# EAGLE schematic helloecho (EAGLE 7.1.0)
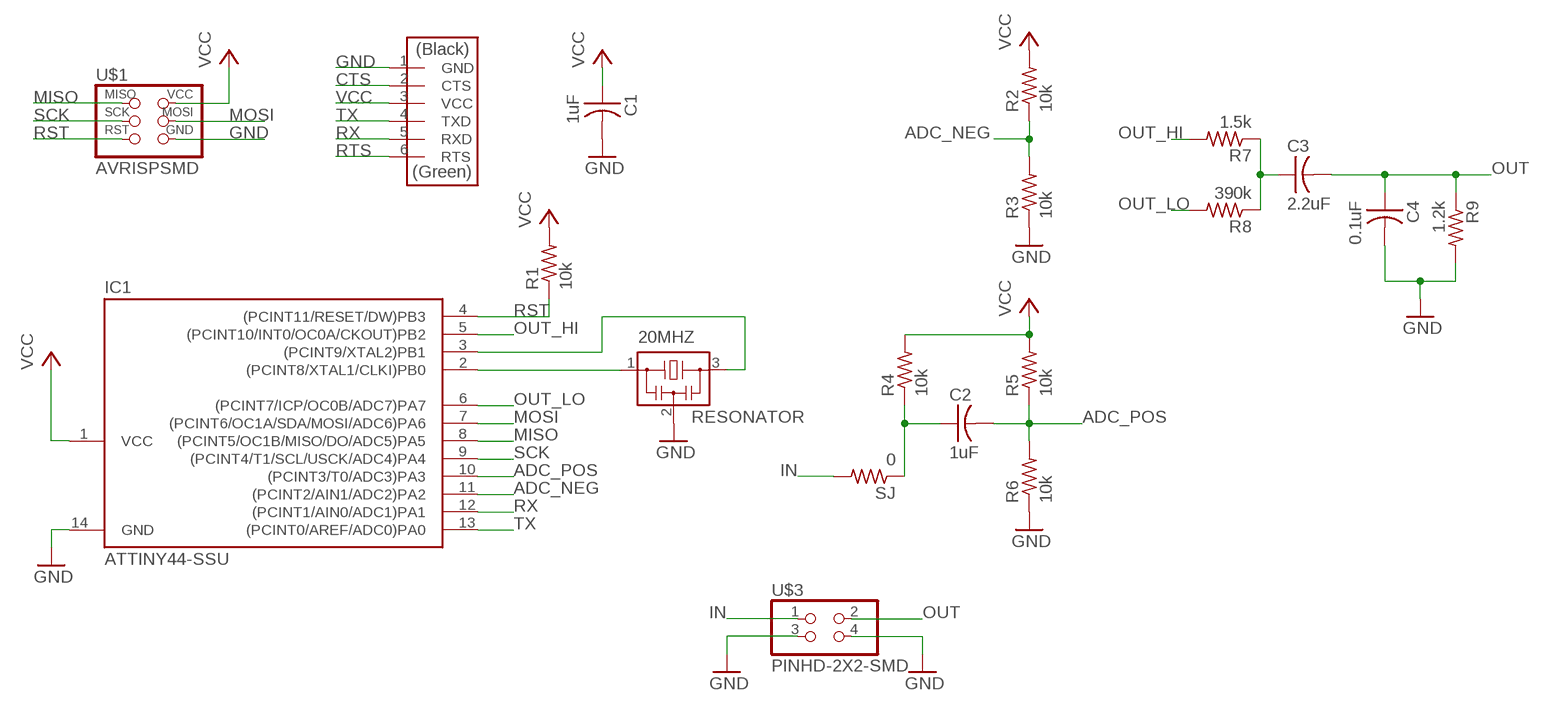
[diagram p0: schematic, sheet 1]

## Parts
20MHZ  RESONATOR  [EFOBM]
C1  1uF  CAP-US1206  [C1206]
C2  1uF  CAP-US1206  [C1206]
C3  2.2uF  CAP-US1206  [C1206]
C4  0.1uF  CAP-US1206  [C1206]
IC1  ATTINY44-SSU  [SOIC14]
R1  10k  RES-US1206  [R1206]
R2  10k  RES-US1206  [R1206]
R3  10k  RES-US1206  [R1206]
R4  10k  RES-US1206  [R1206]
R5  10k  RES-US1206  [R1206]
R6  10k  RES-US1206  [R1206]
R7  1.5k  RES-US1206  [R1206]
R8  390k  RES-US1206  [R1206]
R9  1.2k  RES-US1206  [R1206]
SJ  0  RES-US1206  [R1206]
U$1  AVRISPSMD  [2X03SMD]
U$2  FTDI-SMD-HEADER  [1X06SMD]
U$3  PINHD-2X2-SMD  [2X02SMD]

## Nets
ADC_NEG: IC1.11((PCINT2/AIN1/ADC2)PA2) R2.1 R3.2
ADC_POS: C2.2 IC1.10((PCINT3/T0/ADC3)PA3) R5.1 R6.2
CTS: U$2.2(CTS)
GND: 20MHZ.2 C1.2 C4.2 IC1.14(GND) R3.1 R6.1 R9.2 U$1.6(GND) U$2.1(GND) U$3.3 U$3.4
IN: SJ.2 U$3.1
MISO: IC1.8((PCINT5/OC1B/MISO/DO/ADC5)PA5) U$1.1(MISO)
MOSI: IC1.7((PCINT6/OC1A/SDA/MOSI/ADC6)PA6) U$1.4(MOSI)
N$1: 20MHZ.1 IC1.2((PCINT8/XTAL1/CLKI)PB0)
N$2: 20MHZ.3 IC1.3((PCINT9/XTAL2)PB1)
N$3: C2.1 R4.1 SJ.1
N$5: C3.1 R7.1 R8.1
OUT: C3.2 C4.1 R9.1 U$3.2
OUT_HI: IC1.5((PCINT10/INT0/OC0A/CKOUT)PB2) R7.2
OUT_LO: IC1.6((PCINT7/ICP/OC0B/ADC7)PA7) R8.2
RST: IC1.4((PCINT11/RESET/DW)PB3) R1.1 U$1.5(RST)
RTS: U$2.6(RTS)
RX: IC1.12((PCINT1/AIN0/ADC1)PA1) U$2.5(RXD)
SCK: IC1.9((PCINT4/T1/SCL/USCK/ADC4)PA4) U$1.3(SCK)
TX: IC1.13((PCINT0/AREF/ADC0)PA0) U$2.4(TXD)
VCC: C1.1 IC1.1(VCC) R1.2 R2.2 R4.2 R5.2 U$1.2(VCC) U$2.3(VCC)

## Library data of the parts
20MHZ = fab:RESONATOR
C1-C4 = fab:CAP-US
IC1 = fab:ATTINY44
R1-R9 SJ = fab:RES-US: Resistor (US Symbol)
U$1 = fab:AVRISP
U$2 = fab:FTDI-SMD-HEADER
U$3 = fab:PINHD-2X2-SMD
